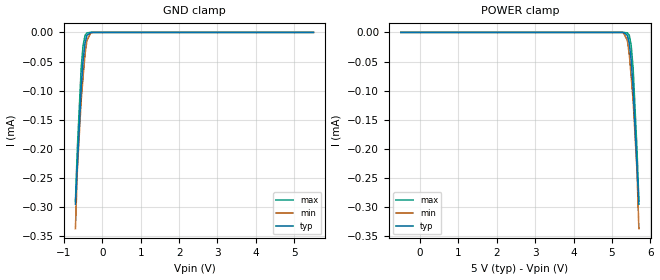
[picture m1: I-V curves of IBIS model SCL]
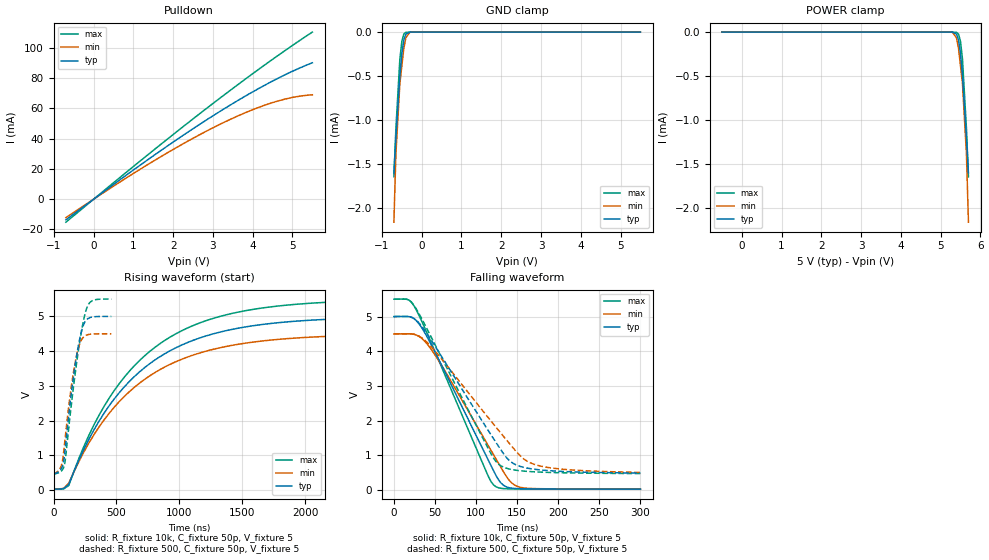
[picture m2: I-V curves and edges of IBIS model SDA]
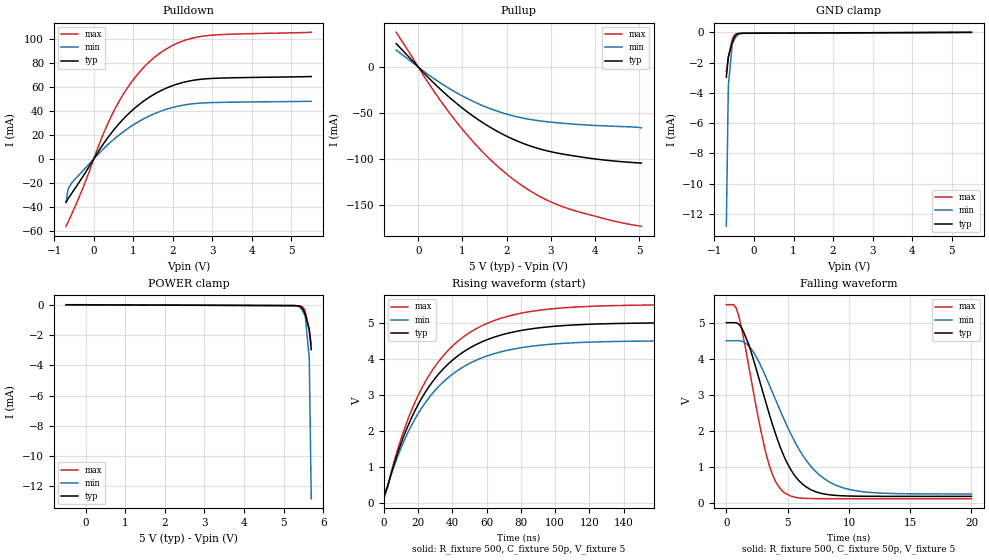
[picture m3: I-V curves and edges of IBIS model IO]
| PCA9538 - IBIS model
[IBIS Ver]   3.2
[Comment Char]   |_char
| VDD nom: 5v; min: 4.5v; max: 5.5v
[File name]   pca9538_5v.ibs
[File Rev]   1
[Date]   Aug 18, 2008 11:26:38 AM
[Source]
[Notes]
[Disclaimer]
(C) Copyright 2007 NXP Semiconductors
All rights reserved
NXP Semiconductors (NXP) does not warrant that this model and any other
accompanying information (Model) accurately or fully represents the
operating characteristics and specifications of the semiconductor
products to which the Model relates.  Moreover, the Model is furnished
on an "as is" and with "all faults" basis, and without support or
warranty of any kind.  NXP disclaims all warranties, whether expressed
or implied or statutory, including without limitation all implied
warranties of non-infringement, merchantability and fitness for any
purpose, and those arising from a course of dealing or usage of trade.
NXP does not convey any license under its or any third party's patents,
copyrights or other intellectual property or proprietary rights.
You and your company assume any and all risks and liability arising out
of the application or use of the Model.
In no event shall NXP be liable for any direct, indirect, special,
consequential or incidental damages, however caused, whether in
warranty, contract or tort (including negligence), strict liability or
other legal theory, including, without limitation, for lost profits,
business interruption, or corruption or loss of data or information,
arising out of or in connection with the use of or the inability to use
the Model, even if NXP has been advised of the possibility of such
damages.
NXP provides the Model as a courtesy to our customers. You and your
company shall not distribute, convey, sell, or give the Model to anyone
else without receiving prior written permission from NXP.
NXP reserves the right to make changes without notice to the Model to
improve reliability, function, or design.
Please be aware that your receipt and subsequent use of the Model shall
serve as acceptance of these terms and conditions.  If you do not
accept these terms, return or destroy the Model immediately.
[Copyright]
2008
| TSSOP16
[Component]   PCA9633PW
Si_location Pin
Timing_location Pin
[Manufacturer]   NXP Semiconductors
[Package]
R_pkg   3.92e-02   3.52e-02   4.56e-02
L_pkg   1.94n   1.65n   2.4n
C_pkg   0.446p   0.335p   0.771p
[Pin] signal_name   model_name   R_pin   L_pin   C_pin
1   A0   Addr   3.52E-02  2.40E-09  0.436E-12
2   A1   Addr   3.70E-02  1.93E-09  0.438E-12
3   RESETb   RESETb   4.56E-02  1.76E-09  0.345E-12
4   IO0   IO   4.00E-02  1.65E-09  0.335E-12
5   IO1   IO   4.00E-02  1.65E-09  0.335E-12
6   IO2   IO   4.56E-02  1.76E-09  0.345E-12
7   IO3   IO   3.70E-02  1.93E-09  0.438E-12
8   Vss   GND   3.52E-02  2.40E-09  0.452E-12
9   IO4   IO   3.52E-02  2.40E-09  0.452E-12
10   IO5   IO   3.70E-02  1.93E-09  0.438E-12
11   IO6   IO   4.56E-02  1.76E-09  0.345E-12
12   IO7   IO   4.00E-02  1.65E-09  0.771E-12
13   INTb   INT_OUT   4.00E-02  1.65E-09  0.771E-12
14   SCL   SCL   4.56E-02  1.76E-09  0.345E-12
15   SDA   SDA   3.70E-02  1.93E-09  0.438E-12
16   VDD   POWER   3.52E-02  2.40E-09  0.452E-12
| SO16
[Component]   PCA9633D16
Si_location Pin
Timing_location Pin
[Manufacturer]   NXP Semiconductors
[Package]
R_pkg   4.96e-02   3.94e-02   5.98e-02
L_pkg   2.52n   1.87n   3.16n
C_pkg   0.628p   0.494p   0.763p
[Pin] signal_name   model_name   R_pin   L_pin   C_pin
1   A0   Addr   5.98E-02  3.16E-09  7.63E-13
2   A1   Addr   4.55E-02  2.41E-09  6.04E-13
3   RESETb   RESETb   4.64E-02  1.93E-09  5.15E-13
4   IO0   IO   3.94E-02  1.87E-09  4.94E-13
5   IO1   IO   3.94E-02  1.87E-09  4.94E-13
6   IO2   IO   4.64E-02  1.93E-09  5.15E-13
7   IO3   IO   4.55E-02  2.41E-09  6.04E-13
8   Vss   GND   5.98E-02  3.16E-09  7.63E-13
9   IO4   IO   5.98E-02  3.16E-09  7.63E-13
10   IO5   IO   4.55E-02  2.41E-09  6.04E-13
11   IO6   IO   4.64E-02  1.93E-09  5.15E-13
12   IO7   IO   3.94E-02  1.87E-09  4.94E-13
13   INTb   INT_OUT   3.94E-02  1.87E-09  4.94E-13
14   SCL   SCL   4.64E-02  1.93E-09  5.15E-13
15   SDA   SDA   4.55E-02  2.41E-09  6.04E-13
16   VDD   POWER   5.98E-02  3.16E-09  7.63E-13
[Define Package Model]  HVQFN16
[Manufacturer]  ST-NXP Wireless
[OEM]  Unknown
[Description]  Full package model
|[Simulated] Chris Hunat
|[Approved] Wayne Nunn, Roger Real
[Number Of Pins]  16
[Pin Numbers]
|Pin Num   Terminal Name
1   | lead1:pin1
2   | lead2:pin2
3   | lead3:pin3
4   | lead4:pin4
5   | lead5:pin5
6   | lead6:pin6
7   | lead7:pin7
8   | lead8:pin8
9   | lead9:pin9
10   | lead10:pin10
11   | lead11:pin11
12   | lead12:pin12
13   | lead13:pin13
14   | lead14:pin14
15   | lead15:pin15
16   | lead16:pin16
[Model Data]
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[End Model Data]
[End Package Model]
| Models and submodels in the file (6): SCL (Input), SDA (I/O_open_drain), IO (I/O), RESETb (Input), INT_OUT (Open_drain), Addr (Input)
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[Model]   SCL
Model_type Input
Vinh=3.5
Vinl=1.5
C_comp   1.84p   1.81p   1.86p
[Temperature Range] 27   85   -40
[Voltage Range]   5   4.5   5.5
[GND Clamp]
-700mV    -295uA     -337uA     -289.5uA
-650mV    -228.6uA   -236.2uA   -199.5uA
-550mV    -96.13uA   -116.2uA   -61.46uA
-500mV    -48.62uA   -75.94uA   -22.35uA
-450mV    -18.67uA   -37.44uA   -5.001uA
-400mV    -4.926uA   -13.83uA   -710.6nA
-300mV    -138.4nA   -722.3nA   -7.551nA
5.5V      13.38pA    37.84pA    11.03pA
[POWER Clamp]
-500mV    13.38pA    37.84pA    11.03pA
5.3V      -138.4nA   -722.3nA   -7.551nA
5.4V      -4.926uA   -13.83uA   -710.6nA
5.45V     -18.67uA   -37.44uA   -5.001uA
5.5V      -48.62uA   -75.94uA   -22.35uA
5.55V     -96.13uA   -116.2uA   -61.46uA
5.65V     -228.6uA   -236.2uA   -199.5uA
5.7V      -295uA     -337uA     -289.5uA
[Model]   SDA
Model_type I/O_open_drain
Enable Active-High
Vinh=3.5
Vinl=1.5
Vref=5
Vmeas=2.5
Rref=10k
Cref=50p
C_comp   6.2p   6p   6.4p
[Temperature Range] 27   85   -40
[Voltage Range]   5   4.5   5.5
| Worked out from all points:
|   slope of the pulldown table from 0 to 0.75 V, typ, clamps not added: 51.6 ohm
|   GND clamp passes 1 mA (typ) near -0.62 V on its own axis
|   falling waveform, R_fixture 10k, C_fixture 50p, V_fixture 5: 20-80 % time 62.1ns typ, 65.9ns min, 59.3ns max; typ from 5 V to 0.027 V
|   falling waveform, R_fixture 500, C_fixture 50p, V_fixture 5: 20-80 % time 72.3ns typ, 81.1ns min, 65ns max; typ from 5 V to 0.49 V
|   rising waveform, R_fixture 10k, C_fixture 50p, V_fixture 5: 20-80 % time 701ns typ, 702ns min, 700ns max; typ from 0.025 V to 5 V
|   rising waveform, R_fixture 500, C_fixture 50p, V_fixture 5: 20-80 % time 96.2ns typ, 87.2ns min, 107ns max; typ from 0.465 V to 5 V
[Pulldown]
-700mV    -13.67mA   -12.19mA   -15.2mA
550mV     10.7mA     9.465mA    11.94mA
1.45V     27.71mA    24.29mA    31.18mA
2.3V      43.07mA    37.33mA    48.94mA
3.1V      56.72mA    48.46mA    65.21mA
3.8V      67.86mA    56.95mA    79.03mA
4.45V     77.33mA    63.37mA    91.43mA
5V        84.48mA    67.19mA    101.5mA
5.5V      90.09mA    68.95mA    110.4mA
[GND Clamp]
-700mV    -1.597mA   -2.155mA   -1.641mA
-650mV    -1.199mA   -1.383mA   -1.095mA
-550mV    -495.5uA   -583.4uA   -306.2uA
-500mV    -240.9uA   -381.2uA   -104.9uA
-450mV    -89.14uA   -184.4uA   -22.18uA
-400mV    -22.76uA   -66.22uA   -3.012uA
-300mV    -607.3nA   -3.323uA   -29.64nA
5.5V      40.19pA    130.8pA    33.06pA
[POWER Clamp]
-500mV    40.19pA    130.8pA    33.06pA
5.3V      -607.3nA   -3.323uA   -29.64nA
5.4V      -22.76uA   -66.22uA   -3.012uA
5.45V     -89.14uA   -184.4uA   -22.18uA
5.5V      -240.9uA   -381.2uA   -104.9uA
5.55V     -495.5uA   -583.4uA   -306.2uA
5.65V     -1.199mA   -1.383mA   -1.095mA
5.7V      -1.597mA   -2.155mA   -1.641mA
[Falling Waveform]
R_fixture=10k
C_fixture=50p
V_fixture=5
V_fixture_min=4.5
V_fixture_max=5.5
0s        5V         4.5V       5.5V
18.18ns   4.999V     4.503V     5.477V
33.33ns   4.697V     4.382V     4.894V
54.55ns   3.765V     3.728V     3.738V
115.2ns   850.2mV    1.268V     383.6mV
121.2ns   561.7mV    1.021V     150.8mV
133.3ns   138.6mV    529.9mV    42.27mV
142.4ns   58.26mV    227.4mV    34.12mV
154.5ns   38.97mV    76.16mV    31.04mV
300ns     26.91mV    28.28mV    25.97mV
[Falling Waveform]
R_fixture=500
C_fixture=50p
V_fixture=5
V_fixture_min=4.5
V_fixture_max=5.5
0s        5V         4.5V       5.5V
15.15ns   5.003V     4.503V     5.5V
24.24ns   4.948V     4.489V     5.331V
48.48ns   4.207V     4.05V      4.265V
118.2ns   1.594V     1.989V     1.049V
130.3ns   1.156V     1.636V     697.9mV
145.5ns   764.9mV    1.205V     583.3mV
157.6ns   656.8mV    906.5mV    547.8mV
172.7ns   594.9mV    727.4mV    523.5mV
300ns     489.7mV    510.6mV    475.8mV
[Rising Waveform]
R_fixture=10k
C_fixture=50p
V_fixture=5
V_fixture_min=4.5
V_fixture_max=5.5
0s        25.37mV    25.7mV     25.12mV
121.2ns   162.6mV    197.2mV    131.5mV
242.4ns   1.183V     1.105V     1.265V
363.6ns   1.994V     1.826V     2.167V
606.1ns   3.137V     2.842V     3.435V
848.5ns   3.846V     3.472V     4.221V
1.172us   4.39V      3.957V     4.825V
1.535us   4.703V     4.235V     5.171V
2.061us   4.895V     4.406V     5.384V
4us       4.997V     4.498V     5.497V
[Rising Waveform]
R_fixture=500
C_fixture=50p
V_fixture=5
V_fixture_min=4.5
V_fixture_max=5.5
0s        465.5mV    467.6mV    463.7mV
60.4ns    606.7mV    690.4mV    543mV
88.28ns   1.031V     1.35V      742.7mV
130.1ns   2.43V      2.672V     2.086V
167.3ns   3.476V     3.576V     3.214V
199.8ns   4.201V     4.114V     4.068V
237ns     4.741V     4.401V     4.854V
264.8ns   4.911V     4.466V     5.243V
297.4ns   4.975V     4.49V      5.427V
460ns     5V         4.5V       5.5V
[Ramp]
R_load=500
dV/dt_r   1.769E+0/6.440E-8   1.721E+0/6.204E-8   1.801E+0/6.654E-8
dV/dt_f   1.737E+0/1.304E-7   1.574E+0/1.747E-7   1.791E+0/9.775E-8
|[End   SDA
[Model]   IO
Model_type I/O
Polarity Non-Inverting
Vinh=3.5
Vinl=1.5
Vref=5
Vmeas=2.5
Rref=500
Cref=50p
C_comp   8p   7.8p   8.2p
[Temperature Range] 27   85   -40
[Voltage Range]   5   4.5   5.5
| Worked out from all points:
|   slope of the pulldown table from 0 to 0.75 V, typ, clamps not added: 22.5 ohm
|   slope of the pullup table from 0 to 0.75 V, typ, clamps not added: 21.6 ohm
|   GND clamp passes 1 mA (typ) near -0.58 V on its own axis
|   falling waveform, R_fixture 500, C_fixture 50p, V_fixture 5: 20-80 % time 2.75ns typ, 3.68ns min, 1.89ns max; typ from 5 V to 0.185 V
|   rising waveform, R_fixture 500, C_fixture 50p, V_fixture 5: 20-80 % time 35.6ns typ, 35.8ns min, 35.5ns max; typ from 0.185 V to 5 V
[Pullup]
-500mV    25.37mA    18.43mA    37.7mA
250mV     -12.46mA   -8.945mA   -18.79mA
800mV     -36.75mA   -26.04mA   -55.57mA
1.05V     -46.38mA   -32.63mA   -70.4mA
1.4V      -58.37mA   -40.62mA   -89.14mA
1.7V      -67.27mA   -46.32mA   -103.4mA
2.05V     -76.08mA   -51.65mA   -117.9mA
2.65V     -87.29mA   -57.63mA   -137.5mA
3.2V      -93.67mA   -60.58mA   -150.1mA
3.55V     -96.46mA   -61.94mA   -155.8mA
4.3V      -101.2mA   -63.91mA   -165.3mA
5.05V     -104.1mA   -65.9mA    -172.6mA
[Pulldown]
-700mV    -36.27mA   -35.86mA   -56.15mA
-650mV    -33.08mA   -25.23mA   -52.69mA
-550mV    -28.29mA   -19.55mA   -45.42mA
-250mV    -13.39mA   -9.024mA   -22.18mA
200mV     10.37mA    6.863mA    17.45mA
550mV     25.85mA    17.44mA    42.41mA
1V        41.2mA     28.31mA    65.93mA
1.25V     47.83mA    33.12mA    75.71mA
1.55V     54.22mA    37.83mA    84.93mA
2.1V      62.15mA    43.65mA    96.11mA
2.7V      66.24mA    46.44mA    101.9mA
5.5V      68.56mA    47.98mA    105.4mA
[GND Clamp]
-700mV    -2.962mA   -12.83mA   -2.603mA
-650mV    -1.632mA   -3.565mA   -1.663mA
-550mV    -661.5uA   -762.3uA   -435.1uA
-500mV    -333uA     -487.6uA   -183.8uA
-450mV    -155.7uA   -258.2uA   -88.16uA
-400mV    -81.62uA   -123.8uA   -63.79uA
-200mV    -51.95uA   -47.06uA   -56.93uA
5.5V      4.991uA    9.99uA     -583.2pA
[POWER Clamp]
-500mV    4.991uA    9.99uA     -583.2pA
5.2V      -51.95uA   -47.06uA   -56.93uA
5.4V      -81.62uA   -123.8uA   -63.79uA
5.45V     -155.7uA   -258.2uA   -88.16uA
5.5V      -333uA     -487.6uA   -183.8uA
5.55V     -661.5uA   -762.3uA   -435.1uA
5.65V     -1.632mA   -3.565mA   -1.663mA
5.7V      -2.962mA   -12.83mA   -2.603mA
[Falling Waveform]
R_fixture=500
C_fixture=50p
V_fixture=5
V_fixture_min=4.5
V_fixture_max=5.5
0s        5V         4.5V       5.5V
808.1ps   4.997V     4.5V       5.403V
1.414ns   4.735V     4.466V     4.558V
2.222ns   3.966V     4.177V     3.064V
3.232ns   2.781V     3.492V     1.375V
3.838ns   2.097V     3.009V     727.3mV
4.646ns   1.342V     2.366V     308.7mV
6.465ns   458mV      1.21V      129mV
9.091ns   207.3mV    472mV      120.1mV
20ns      185mV      250.5mV    120.1mV
[Rising Waveform]
R_fixture=500
C_fixture=50p
V_fixture=5
V_fixture_min=4.5
V_fixture_max=5.5
0s        185mV      250.2mV    120.1mV
10.1ns    1.669V     1.538V     1.799V
16.16ns   2.366V     2.156V     2.578V
22.22ns   2.919V     2.647V     3.194V
28.28ns   3.356V     3.034V     3.68V
36.36ns   3.8V       3.428V     4.172V
52.53ns   4.36V      3.927V     4.794V
70.71ns   4.685V     4.218V     5.154V
96.97ns   4.887V     4.398V     5.376V
200ns     4.998V     4.498V     5.498V
[Ramp]
R_load=500
dV/dt_r   1.841E+0/7.108E-10   1.502E+0/1.182E-9   2.170E+0/3.921E-10
dV/dt_f   1.933E+0/3.122E-10   1.616E+0/5.107E-10   2.241E+0/1.918E-10
|[End   IO
